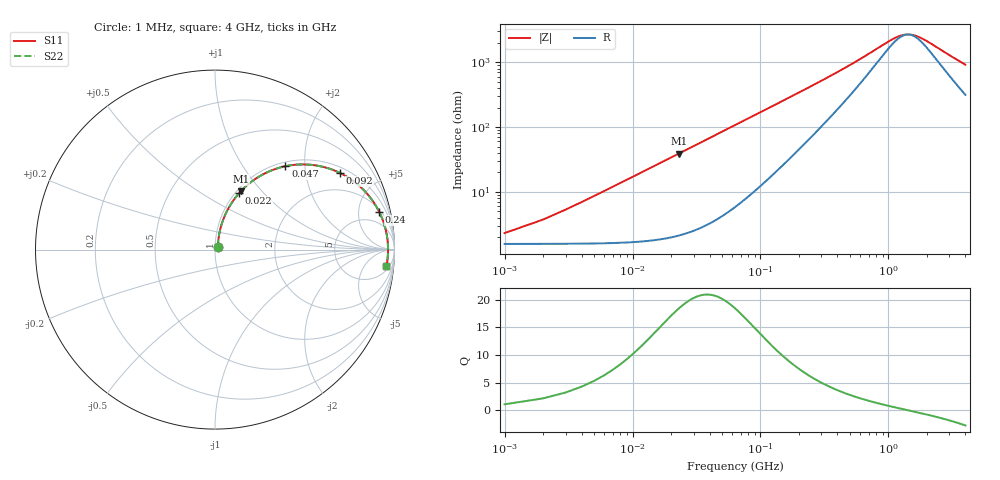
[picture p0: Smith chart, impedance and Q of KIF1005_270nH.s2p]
!version-2
!date-12.2020
!Series
# MHz S RI R 50
!Freq ReS11 ImS11 ReS21 ImS21 ReS12 ImS12 ReS22 ImS22
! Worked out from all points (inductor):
!   4000 points, 1 MHz to 4 GHz, reference 50 ohm
!   read as one part in series: L = 269 nH near 21 MHz
!   highest Q = 18.5 at 23 MHz (marker M1), where L = 269 nH
!   self-resonance near 1.423 GHz
!   S11 on the Smith chart (normalised r, x): 1 MHz: 1.03, +0.03; 22 MHz: 1.04, +0.74; 47 MHz: 1.08, +1.59; 92 MHz: 1.21, +3.11; 240 MHz: 2.30, +8.15; 4 GHz: 7, -17
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1  0.0157 0.0164  0.9843 -0.0164  0.9843 -0.0164  0.0157 0.0164
11  0.0484 0.1739  0.9516 -0.1739  0.9516 -0.1739  0.0484 0.1739
22  0.1349 0.3151  0.8651 -0.3151  0.8651 -0.3151  0.1349 0.3151
23  0.1445 0.3256  0.8555 -0.3256  0.8555 -0.3256  0.1445 0.3256
27  0.1847 0.3636  0.8153 -0.3636  0.8153 -0.3636  0.1847 0.3636
33  0.248 0.4084  0.752 -0.4084  0.752 -0.4084  0.248 0.4084
47  0.3927 0.4646  0.6073 -0.4646  0.6073 -0.4646  0.3927 0.4646
69  0.5734 0.4671  0.4266 -0.4671  0.4266 -0.4671  0.5734 0.4671
92  0.6967 0.4269  0.3033 -0.4269  0.3033 -0.4269  0.6967 0.4269
117  0.7796 0.3755  0.2204 -0.3755  0.2204 -0.3755  0.7796 0.3755
148  0.8405 0.3193  0.1595 -0.3193  0.1595 -0.3193  0.8405 0.3193
240  0.9147 0.2108  0.0853 -0.2108  0.0853 -0.2108  0.9147 0.2108
419  0.9493 0.1179  0.0507 -0.1179  0.0507 -0.1179  0.9493 0.1179
668  0.9599 0.0639  0.0401 -0.0639  0.0401 -0.0639  0.9599 0.0639
1025  0.9635 0.0258  0.0365 -0.0258  0.0365 -0.0258  0.9635 0.0258
1182  0.964 0.0144  0.036 -0.0144  0.036 -0.0144  0.964 0.0144
1334  0.9642 0.00498  0.0358 -0.00498  0.0358 -0.00498  0.9642 0.00498
1595  0.9642 -0.00885  0.0358 0.00885  0.0358 0.00885  0.9642 -0.00885
2001  0.9635 -0.0269  0.0365 0.0269  0.0365 0.0269  0.9635 -0.0269
2667  0.9615 -0.0517  0.0385 0.0517  0.0385 0.0517  0.9615 -0.0517
3334  0.9586 -0.0736  0.0414 0.0736  0.0414 0.0736  0.9586 -0.0736
4000  0.955 -0.094  0.045 0.094  0.045 0.094  0.955 -0.094
